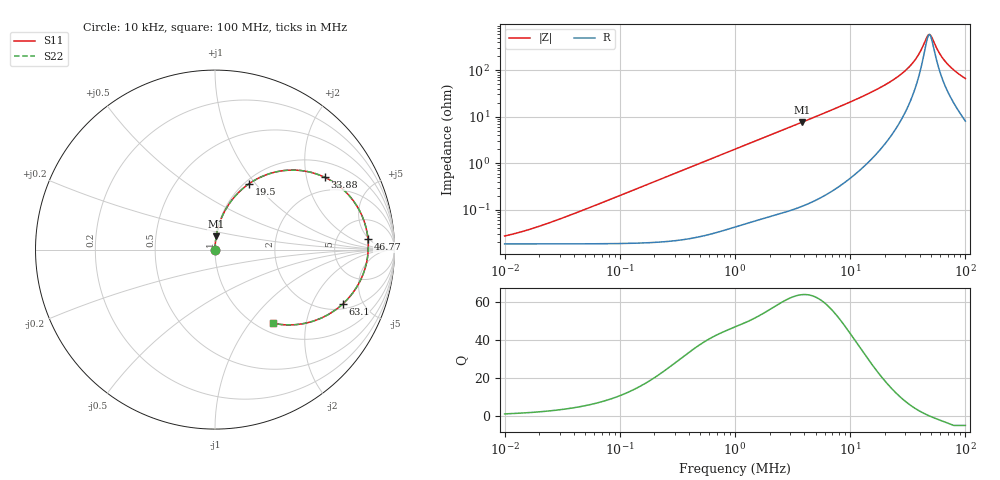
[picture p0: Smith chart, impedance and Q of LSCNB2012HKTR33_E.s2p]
! LSCNB2012HKTR33_E  S-PARAMETER MODEL  ( Standard Model )
! Model Generated by TAIYO YUDEN Corporation (http://www.ty-top.com)
! Version 1.0
! TAIYO YUDEN Control No. 220720
! Copyright(c) 2022 TAIYO YUDEN CO.,LTD. All Rights Reserved.
! Product Description (link to TY-COMPAS)
! https://ds.yuden.co.jp/TYCOMPAS/or/detail?pn=LSCNB2012HKTR33ME&u=M
! Products Name : Inductors
! Characteristics :
!  Inductance : 0.33 [uH] , SRF(min) : - [Hz] , DC Resistance(max) : 25 [mOhm]
!  Rated Current : Saturation  5.4 [A] (dL = 30 [%]), Temp Rise  4.1 [A] (dT = 40 [degC])
!  Case Size : 2.0 x 1.2 / 0.079 x 0.047 [mm/inch] , Thickness : 0.8 / 0.031 [mm/inch]
!  (Conditions: Temperature = 25 [degC] , DC Bias Current = 0 [A])
! External Node Assignments :
!  1  o---GGG---o  2
! GND o---------o GND
! Frequency Range : 10kHz  -  100MHz  [ 402 STEP ]
# MHz S RI R 50
! Freq[MHz].  S11 Real  S11 Imag  S21 Real  S21 Imag  S12 Real  S12 Imag  S22 Real  S22 Imag
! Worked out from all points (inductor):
!   401 points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, 10 kHz to 100 MHz, reference 50 ohm
!   read as one part in series: L = 321 nH near 28.18 kHz
!   highest Q = 63.9 at 3.802 MHz (marker M1), where L = 317 nH
!   self-resonance near 48.75 MHz
!   S11 on the Smith chart (normalised r, x): 10 kHz: 1.00, +0.00; 19.5 MHz: 1.05, +0.92; 33.88 MHz: 1.48, +2.57; 46.77 MHz: 11, +5; 63.1 MHz: 2.29, -3.46; 100 MHz: 1.16, -1.31
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0.01  0.000185 0.000201  0.9998 -0.000201  0.9998 -0.000201  0.000185 0.000201
0.019055  0.000185 0.000384  0.9998 -0.000384  0.9998 -0.000384  0.000185 0.000384
0.046774  0.000187 0.000942  0.9998 -0.000942  0.9998 -0.000942  0.000187 0.000942
0.218776  0.000222 0.0044  0.9998 -0.0044  0.9998 -0.0044  0.000222 0.0044
1  0.000825 0.02  0.9992 -0.02  0.9992 -0.02  0.000825 0.02
3.801894  0.00684 0.075  0.9932 -0.075  0.9932 -0.075  0.00684 0.075
4.677351  0.0101 0.0922  0.9899 -0.0922  0.9899 -0.0922  0.0101 0.0922
11.48154  0.06 0.2247  0.94 -0.2247  0.94 -0.2247  0.06 0.2247
15.48817  0.1134 0.2991  0.8866 -0.2991  0.8866 -0.2991  0.1134 0.2991
19.49845  0.1883 0.3659  0.8117 -0.3659  0.8117 -0.3659  0.1883 0.3659
21.87762  0.2436 0.3987  0.7564 -0.3987  0.7564 -0.3987  0.2436 0.3987
28.18383  0.4261 0.443  0.5739 -0.443  0.5739 -0.443  0.4261 0.443
33.88442  0.6116 0.4029  0.3884 -0.4029  0.3884 -0.4029  0.6116 0.4029
39.81072  0.7704 0.2728  0.2296 -0.2728  0.2296 -0.2728  0.7704 0.2728
46.77351  0.8523 0.0598  0.1477 -0.0598  0.1477 -0.0598  0.8523 0.0598
48.97788  0.8535 -0.00682  0.1465 0.00682  0.1465 0.00682  0.8535 -0.00682
50.11872  0.8503 -0.0397  0.1497 0.0397  0.1497 0.0397  0.8503 -0.0397
57.54399  0.785 -0.2164  0.215 0.2164  0.215 0.2164  0.785 -0.2164
63.09573  0.711 -0.3038  0.289 0.3038  0.289 0.3038  0.711 -0.3038
69.1831  0.6268 -0.3641  0.3732 0.3641  0.3732 0.3641  0.6268 -0.3641
77.62471  0.5207 -0.4061  0.4793 0.4061  0.4793 0.4061  0.5207 -0.4061
100  0.3225 -0.4101  0.6775 0.4101  0.6775 0.4101  0.3225 -0.4101
